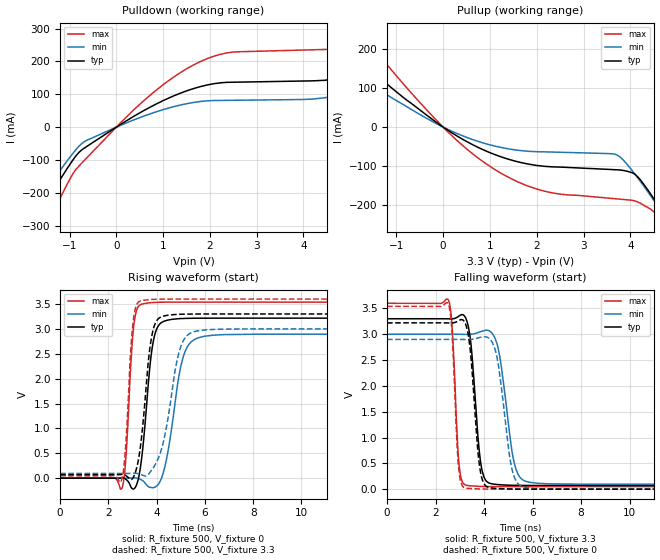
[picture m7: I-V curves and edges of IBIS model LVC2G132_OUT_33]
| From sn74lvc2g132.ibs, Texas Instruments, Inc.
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[Model]   LVC2G132_OUT_33
Model_type  Output
Vref =   0
Rref =   500
Cref =   50p
Vmeas =   1.5
| variable   typ   min   max
C_comp   9.53pF   5.87pF   13.15pF
| C_pullup   9.86pF   5.87pF   11.99pF
| C_pulldown   9.20pF   6.47pF   13.15pF
[Temperature Range]   40   100   -40
| Ambient temperature   25   85   -40
[Voltage range]   3.3   3   3.6
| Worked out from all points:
|   slope of the pulldown table from 0 to 0.495 V, typ, clamps not added: 11.5 ohm
|   slope of the pullup table from 0 to 0.495 V, typ, clamps not added: 13.6 ohm
|   rising waveform, R_fixture 500, V_fixture 0: 20-80 % time 368ps typ, 552ps min, 241ps max; typ from 0 V to 3.22 V
|   falling waveform, R_fixture 500, V_fixture 3.3: 20-80 % time 316ps typ, 477ps min, 208ps max; typ from 3.3 V to 0.07 V
|   rising waveform, R_fixture 500, V_fixture 3.3: 20-80 % time 383ps typ, 619ps min, 245ps max; typ from 0.07 V to 3.3 V
|   falling waveform, R_fixture 500, V_fixture 0: 20-80 % time 309ps typ, 458ps min, 204ps max; typ from 3.22 V to 0 V
[Pulldown]
| LVC2G132_OUT_33
|   Voltage   I(typ)   I(min)   I(max)
-5.5V     -1.107A    -970.8mA   -1.353A
-2.055V   -353.2mA   -300.4mA   -454.5mA
-1.49V    -224.6mA   -188.2mA   -296.4mA
-740mV    -69.5mA    -50.1mA    -109.7mA
365mV     32.28mA    21.63mA    51.56mA
2.22V     134.9mA    81.36mA    221.6mA
4.92V     153.7mA    101.9mA    243.5mA
6.98V     278.6mA    201.4mA    397.7mA
7.35V     308.4mA    129.2mA    438.3mA
7.84V     330.1mA    92.32mA    495.6mA
8.75V     170.7mA    93.06mA    502mA
11V       160mA      96.27mA    278.2mA
[Pullup]
| LVC2G132_OUT_33
|   Voltage   I(typ)   I(min)   I(max)
-5.5V     609.5mA    479.2mA    854.2mA
-3.49V    364.8mA    283mA      516.7mA
-2.685V   271.1mA    208.6mA    386.5mA
-1.96V    190.3mA    144.9mA    273.3mA
-55mV     4.572mA    3.33mA     6.783mA
1.095V    -70.05mA   -48.34mA   -108.1mA
2.155V    -100.5mA   -63.45mA   -164.1mA
3.69V     -109.4mA   -70.27mA   -184mA
4.135V    -124.9mA   -126.7mA   -191mA
4.79V     -237.5mA   -238.3mA   -272mA
5V        -277.7mA   -275.7mA   -316.9mA
11V       -1.518A    -1.406A    -1.753A
[Ramp]
| LVC2G132_OUT_33
| variable   typ   min   max
dV/dt_r   2.06/4.03E-10   1.85/5.95E-10   2.26/2.65E-10
dV/dt_f   1.98/3.35E-10   1.79/4.97E-10   2.18/2.22E-10
R_load = 500
[Rising Waveform]
| LVC2G132_OUT_33
R_fixture =   500
C_fixture =   0
L_fixture =   0
V_fixture =   0
V_fixture_min = 0
V_fixture_max = 0
|   Time   V(typ)   V(min)   V(max)
0s        144.1pV    5.487nV    2.182nV
2.565ns   6.264mV    -185.1uV   -198.6mV
2.725ns   -22.33mV   -553.9uV   408.5mV
3.05ns    -217.7mV   6.463mV    3.05V
3.46ns    763.3mV    -64.1mV    3.507V
3.76ns    2.417V     -186.1mV   3.527V
4.02ns    3.018V     -150.7mV   3.535V
5.12ns    3.21V      2.463V     3.539V
6.01ns    3.216V     2.854V     3.539V
40ns      3.216V     2.894V     3.539V
[Falling Waveform]
| LVC2G132_OUT_33
R_fixture =   500
C_fixture =   0
L_fixture =   0
V_fixture =   3.3
V_fixture_min = 3
V_fixture_max = 3.6
|   Time   V(typ)   V(min)   V(max)
0s        3.3V       3V         3.6V
2.535ns   3.298V     3V         3.66V
2.69ns    3.298V     3V         3.102V
2.97ns    3.353V     2.999V     481.2mV
3.3ns     3.244V     2.997V     71.54mV
3.87ns    490mV      3.052V     53.56mV
4.315ns   104.5mV    3.029V     49.98mV
5.27ns    74.37mV    464.4mV    48.61mV
5.895ns   71.59mV    132mV      48.51mV
40ns      70.49mV    94.56mV    48.41mV
[Rising Waveform]
| LVC2G132_OUT_33
R_fixture =   500
C_fixture =   0
L_fixture =   0
V_fixture =   3.3
V_fixture_min = 3
V_fixture_max = 3.6
|   Time   V(typ)   V(min)   V(max)
0s        70.47mV    94.51mV    48.4mV
2.51ns    72.78mV    94.43mV    -82.29mV
2.695ns   59.26mV    94.03mV    502.1mV
3.025ns   9.142mV    100.1mV    3.131V
3.365ns   779mV      68.84mV    3.568V
3.7ns     2.534V     101.1mV    3.588V
3.955ns   3.123V     284mV      3.596V
4.975ns   3.294V     2.606V     3.6V
5.725ns   3.299V     2.963V     3.6V
40ns      3.3V       3V         3.6V
[Falling Waveform]
| LVC2G132_OUT_33
R_fixture =   500
C_fixture =   0
L_fixture =   0
V_fixture =   0
V_fixture_min = 0
V_fixture_max = 0
|   Time   V(typ)   V(min)   V(max)
0s        3.22V      2.9V       3.542V
2.53ns    3.219V     2.9V       3.585V
2.68ns    3.218V     2.9V       3.027V
2.95ns    3.262V     2.9V       431.6mV
3.23ns    3.207V     2.898V     18.72mV
3.82ns    433.7mV    2.937V     4.604mV
4.22ns    29.32mV    2.917V     1.577mV
5.165ns   3.157mV    364.7mV    217.3uV
5.72ns    999.4uV    31.69mV    111.3uV
40ns      24.71uV    37.09uV    14.02uV
